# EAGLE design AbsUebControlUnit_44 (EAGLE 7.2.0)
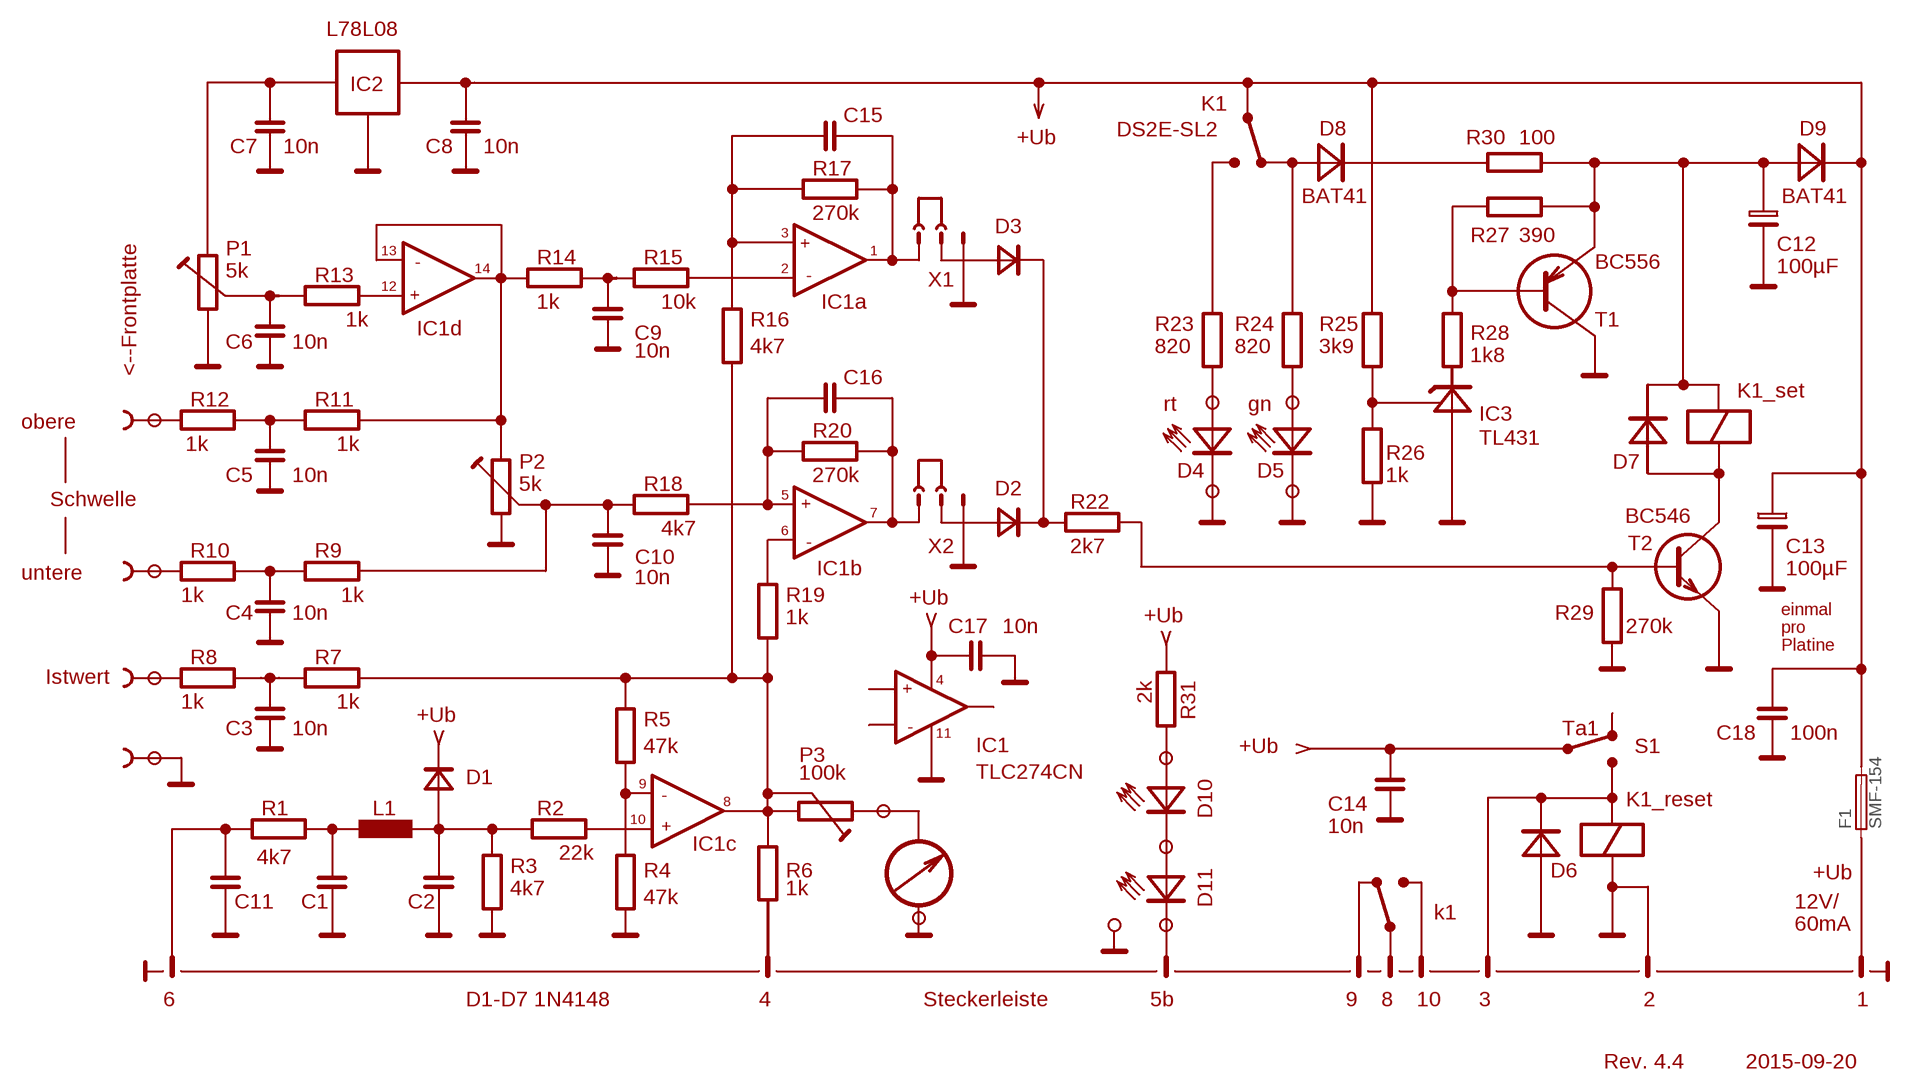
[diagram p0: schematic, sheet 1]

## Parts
F1  SMF-154  [SMF-154]
Unconnected: F1.1 F1.2

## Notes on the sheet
- L78L08
- IC2
- K1
- C15
- DS2E-SL2 | D8 | D9
- +Ub | R30 | 100
- C7 | 10n | C8 | 10n
- R17
- BAT41 | BAT41
- 270k
- D3
- 3 | +
- R27 | 390
- P1 | C12
- 13 | - | 1
- R14 | R15 | - | BC556
- 14 | 2 | 100µF
- 5k | R13
- X1
- 12
- +
- 1k | 10k | IC1a
- 1k | R16 | R23 | R24 | R25 | T1
- IC1d | C9 | R28
- C6 | 10n | 4k7 | 820 | 820 | 3k9
- 10n | 1k8
- <--Frontplatte
- C16
- K1_set
- R12 | R11 | rt | gn
- IC3
- obere
- R20
- TL431
- 1k | 1k
- R26
- P2 | D7
- C5 | 10n | 270k | D4 | D5 | 1k
- Schwelle | 5k | R18 | D2
- 5
- + | R22
- 7
- BC546
- 4k7 | 6 | - | T2
- C10 | X2 | 2k7 | C13
- R10 | R9
- untere | IC1b | 100µF
- 10n
- 1k | 1k | R19 | +Ub
- C4 | 10n | R29 | einmal
- 1k | +Ub
- C17 | 10n | 270k | pro
- Platine
- Istwert | R8 | R7
- 2k | R31
- 4
- +
- 1k | 1k
- +Ub | -
- R5
- C3 | 10n | 11 | Ta1 | C18 | 100n
- 47k | IC1 | +Ub | S1
- P3
- D1 | 100k | TLC274CN | D10
- 9 | -
- 8 | K1_reset
- R1 | L1 | R2 | C14
- +
- 10
- 10n
- IC1c
- 4k7 | 22k | +Ub
- R3 | D11
- R4 | R6 | D6
- 4k7 | 1k
- C11 | C1 | C2 | 47k | k1 | 12V/
- 60mA
- 6 | D1-D7 1N4148 | 4 | Steckerleiste | 5b | 9 | 8 | 10 | 3 | 2 | 1
- Rev. 4.4 | 2015-09-20

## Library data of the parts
F1 = AbsUebParts_11:SMF-154: Littelfuse Surface Mount Fuse; MF: Littelfuse; MPN: 154.250; OC_REICHELT: SMD-HASF 0,25A; OC_RS: 219-6068

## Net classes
0 default: clearance 0.205 mm

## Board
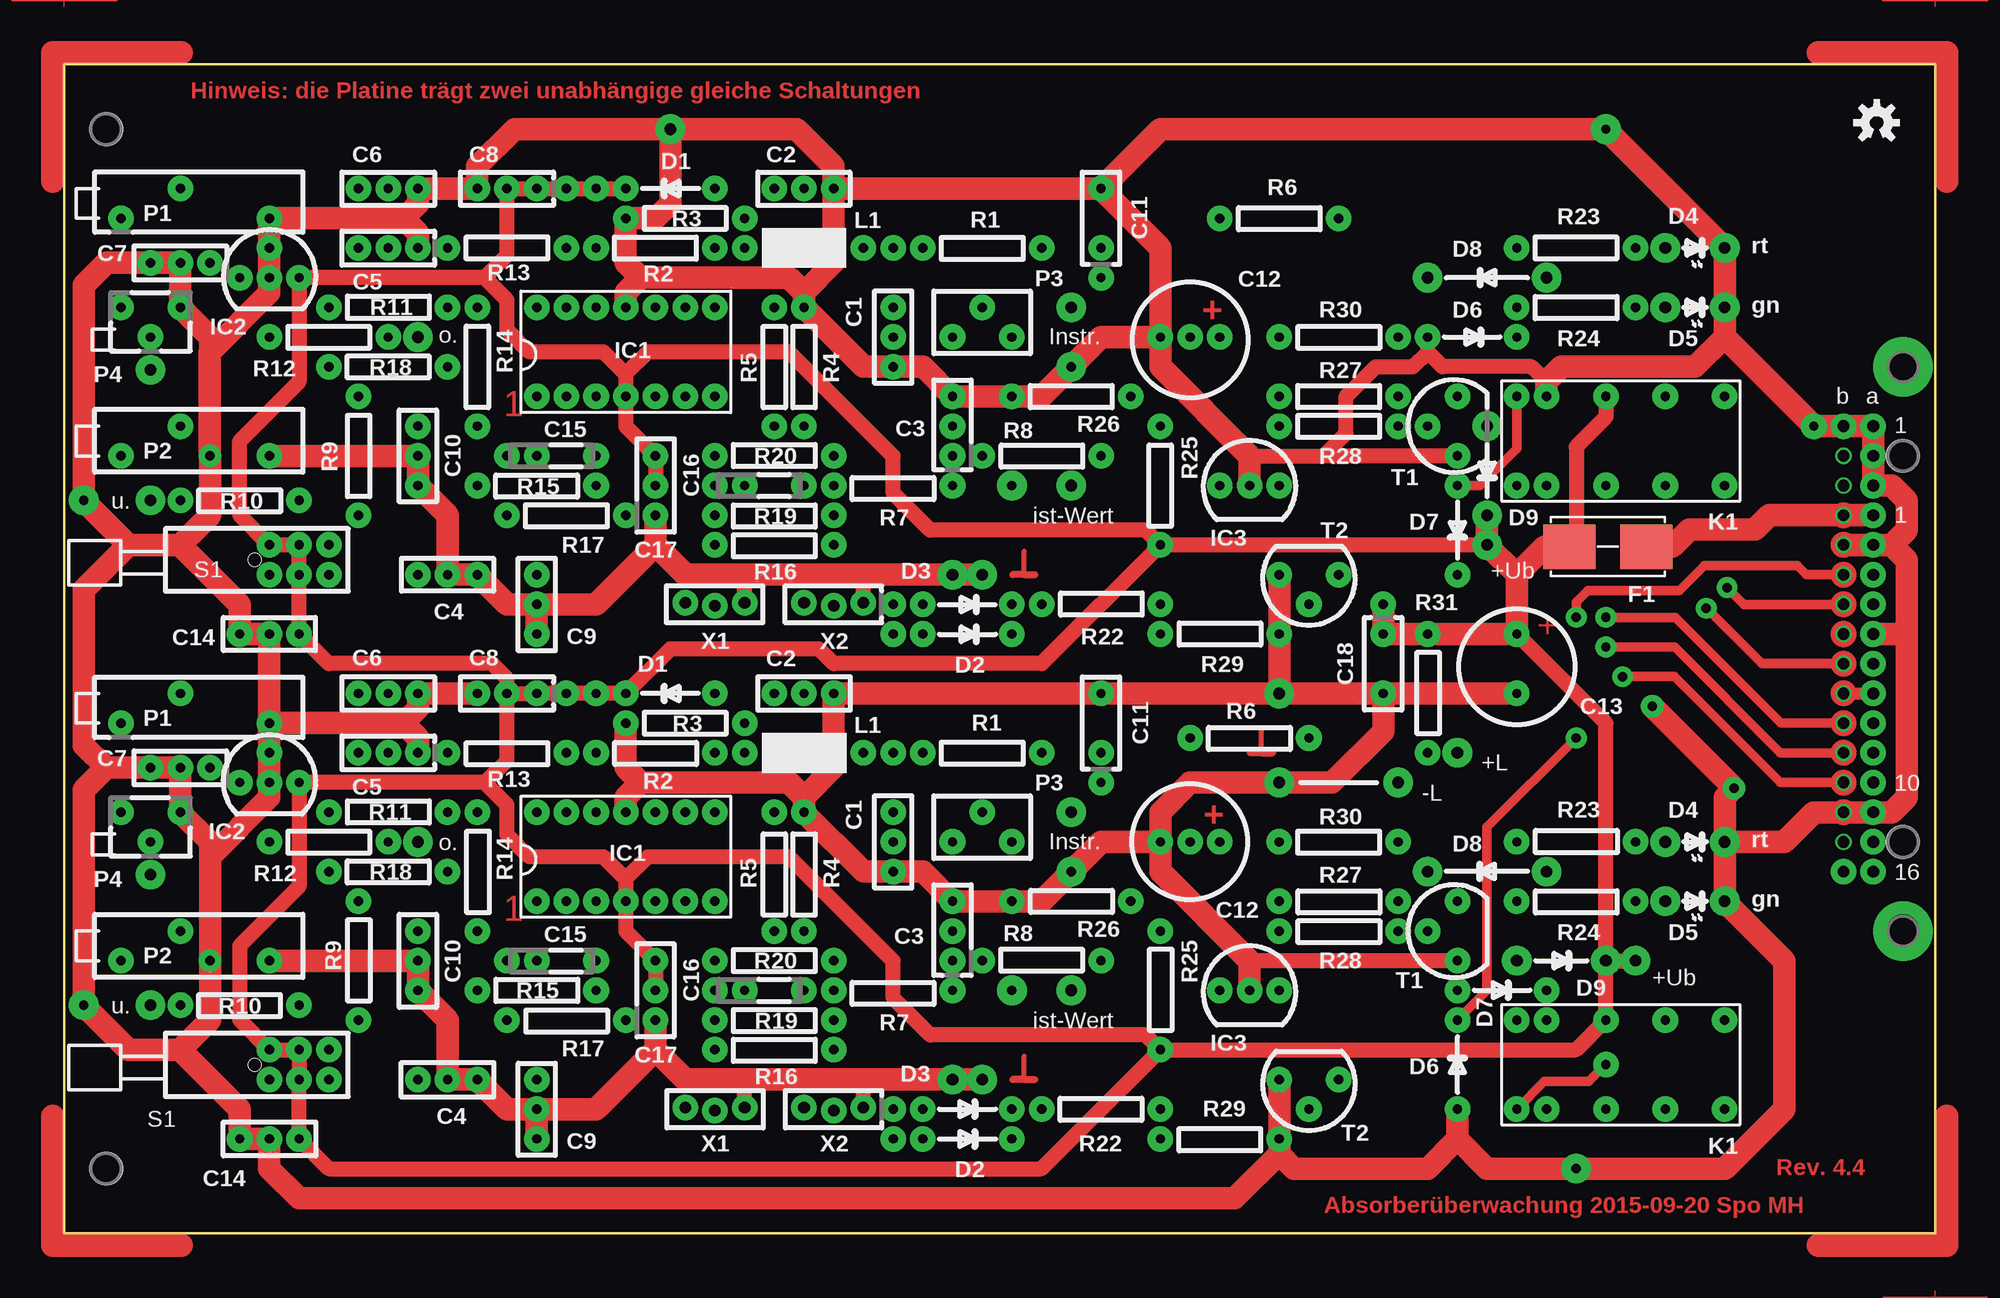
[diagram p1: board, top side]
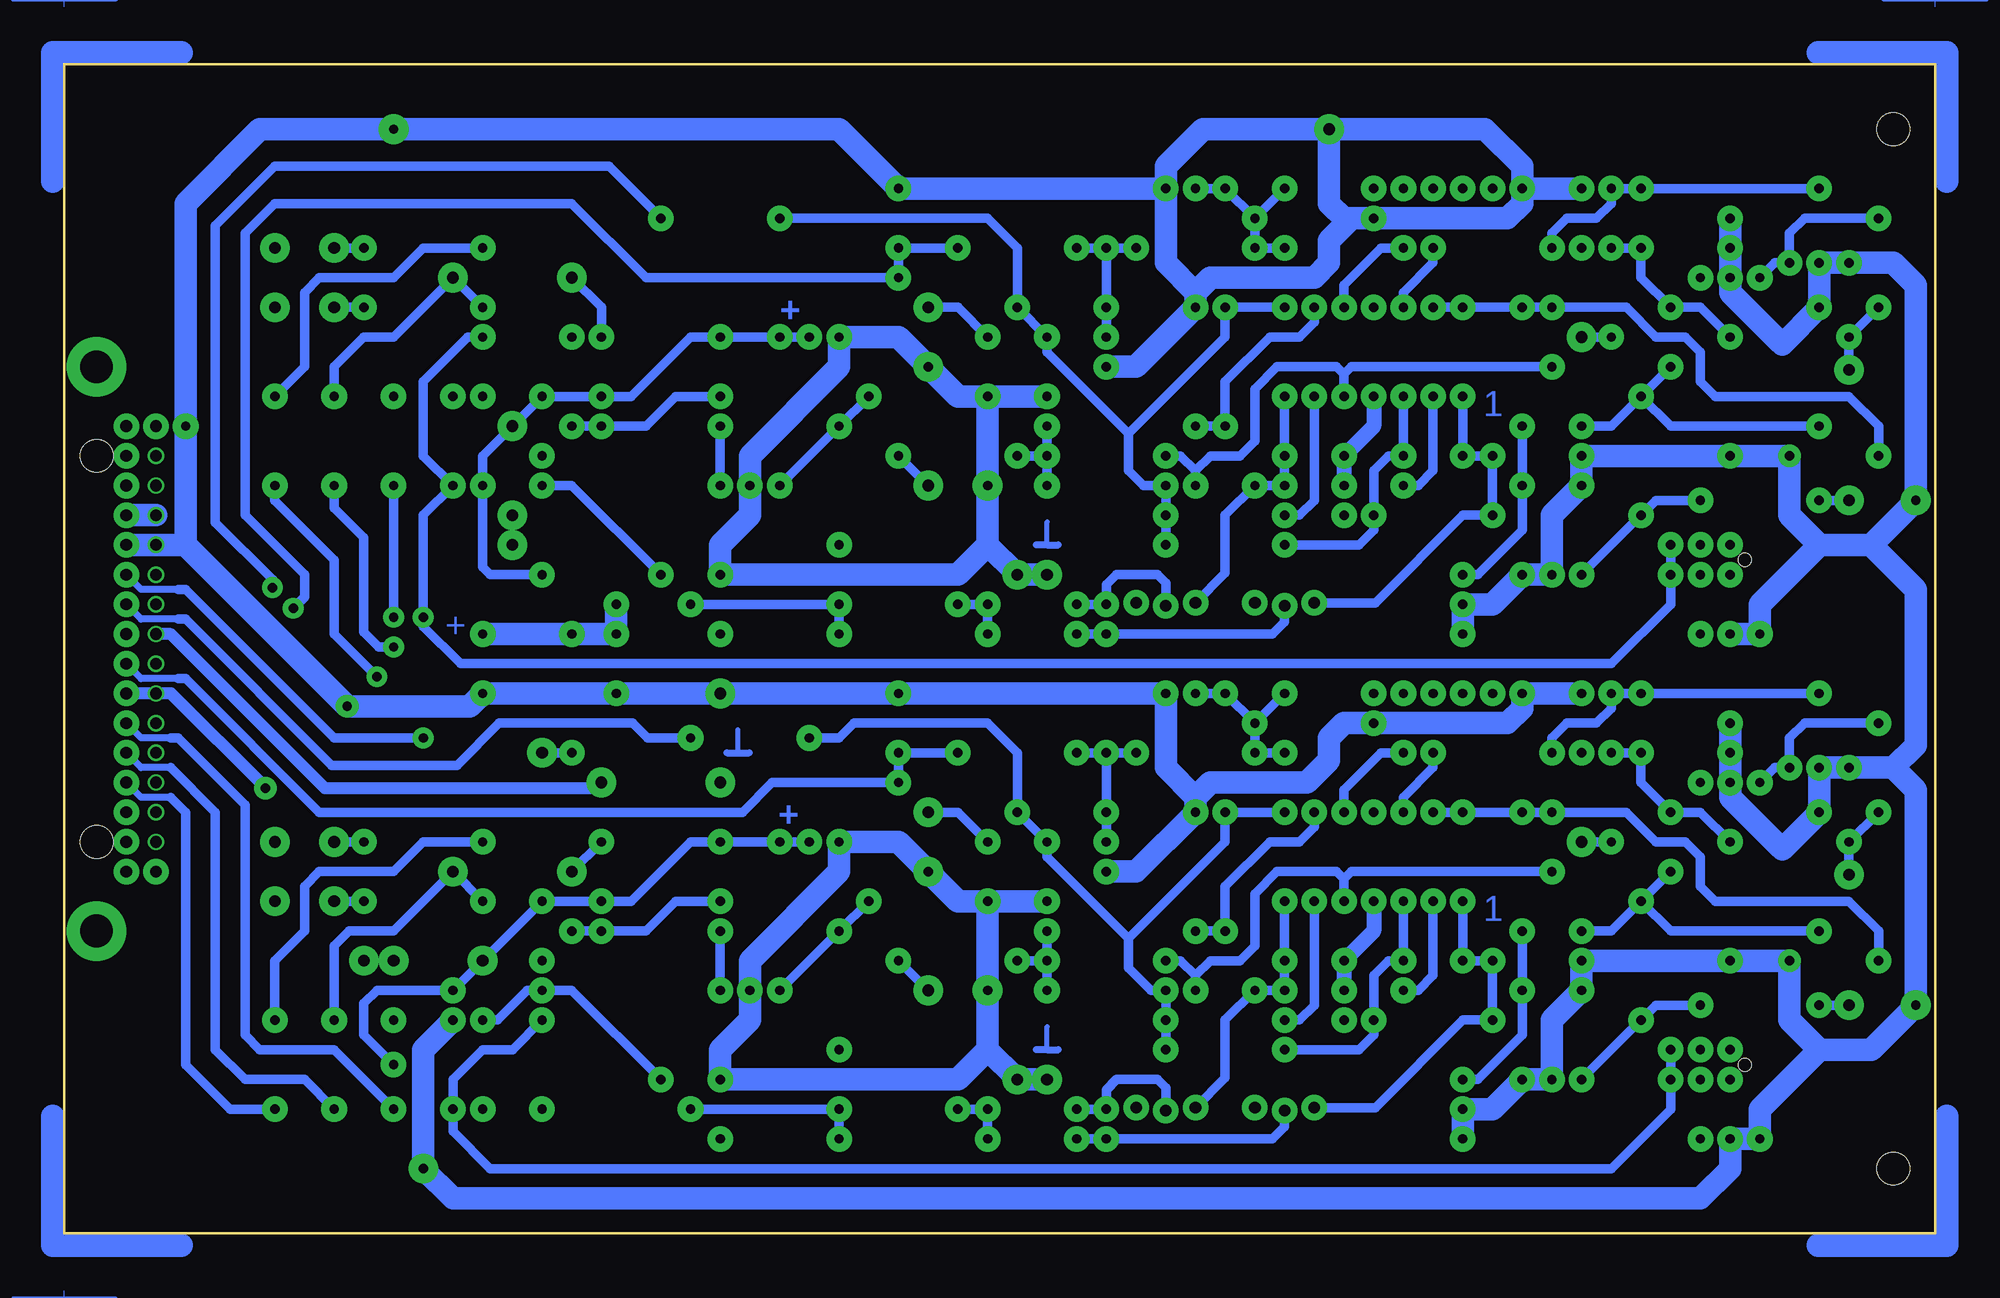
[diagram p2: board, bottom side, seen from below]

Size 160 x 100 mm. Coordinates in mm from the lower left corner, seen from the top.
Outline: 0,0 160,0 160,100 0,100 0,0
Copper layers (1*16): Top 0.035mm / dielectric 1.5mm / Bottom 0.035mm
Design rules "Aetzwerk-DRC 2 Lagen 35µm Cu": minimum track width 6mil, minimum drill 12mil, track to track 6mil, track to pad 6mil, pad to pad 6mil, via to via 6mil, smd to smd 6mil, copper to edge 20mil, drill to drill 8mil, minimum pad ring 8mil, minimum via ring 6mil, stop-mask expansion 3mil, vias tented up to drill 0mil, thermal gap 8mil
Holes 2.8 mm at 3.57,5.55 3.57,94.45 157.24,33.49 157.24,66.51
Holes 1.1 mm at 16.27,57.62 16.27,14.44
vRestrict: area 1.3,92.2 to 5.9,96.7; area 1.3,3.3 to 5.9,7.8; area 155,71.8 to 159.5,76.4; area 155,23.6 to 159.5,28.2

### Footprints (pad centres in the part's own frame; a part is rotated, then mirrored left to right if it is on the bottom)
SMF-154 = smd 4.445 x 3.81: 1 -3.289,0; 2 3.289,0

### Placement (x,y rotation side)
DRILEGEND  [DRILEGEND]  not placed on the board
F1  132,58.74 0 top
PM1  [PASSMARK]  not placed on the board
PM2  [PASSMARK]  not placed on the board
PM3  [PASSMARK]  not placed on the board

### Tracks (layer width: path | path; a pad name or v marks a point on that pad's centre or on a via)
+L  (via drill 0.8 pad 2.18, 1 pad 2.54)
  Bottom 0.813: v116.6,41.11 v119.14,41.11
+UB  (via drill 1 pad 1.4, 1 pad 2.18)
  Top 1.93: v154.7,61.43 v152.16,61.43 145.81,61.43 144.57,60.2 138.96,60.2 137.5,58.74 135.19,58.74
  Bottom 1.93: v152.16,61.43 v154.7,61.43
-L  (via drill 1 pad 1.4, 1 pad 2.54)
  Bottom 1.016: v152.16,51.27 150.89,51.27 137.72,38.1 114.53,38.1 v114.06,38.57
GND  (via drill 0.8 pad 1.93, 0.8 pad 2.18, 0.8 pad 2.54, 1 pad 1.4, 1 pad 2.18, 1 pad 2.54)
  Top 0.813: 58.18,13.17 58.42,13.17
  Top 1.016: v152.16,46.19 v154.7,46.19 | 157.56,51.27 157.56,50.8
  Top 1.27: 116.6,75.4 v116.6,76.67 | 116.6,75.4 117.87,74.13 125.49,74.13 126.76,72.86 | 116.6,75.4 115.33,74.13 112.16,74.13 109.61,71.59 109.61,68.42 107.71,66.51 | 101.36,66.51 107.71,66.51 | v119.14,66.51 107.71,66.51 | v119.14,23.33 101.36,23.33 | v58.18,10.76 58.18,13.17 | v68.34,10.76 68.34,13.17 68.58,13.17 | v58.18,53.94 58.18,56.35 58.42,56.35 | v68.34,53.94 68.34,56.35 67.94,56.35
  Top 1.93: 119.14,8.09 v119.14,10.63 | 119.14,8.09 121.68,5.55 v129.3,5.55 142,5.55 147.08,10.63 147.08,23.33 v142,28.41 v142,33.49 | 119.14,8.09 116.6,5.55 105.17,5.55 103.9,6.82 | v40.4,10.63 v40.4,8.09 | v126.76,71.59 126.76,72.86 128.03,74.13 139.46,74.13 142,76.67 | v101.36,20.79 101.36,23.33 93.74,30.95 v93.74,33.49 | 50.56,15.71 v50.56,18.25 | 50.56,15.71 53.1,13.17 58.42,13.17 68.58,13.17 v75.96,13.17 v78.5,13.17 | 103.9,6.82 v103.9,8.09 v103.9,13.17 | 156.29,58.89 157.56,60.16 157.56,62.7 156.29,63.97 v154.7,63.97 v154.7,66.51 v154.7,69.05 v152.16,69.05 v149.62,69.05 142,76.67 | 156.29,58.89 157.56,57.62 157.56,50.8 157.56,37.3 156.29,36.03 v154.7,36.03 v152.16,36.03 149.62,36.03 147.08,33.49 v142,33.49 | v142,33.49 142,37.3 v142.79,38.09 v135.81,45.08 | 156.29,58.89 v154.7,58.89 v152.16,58.89 | v93.74,33.49 93.74,36.03 96.28,38.57 v103.9,38.57 108.42,38.57 112.79,42.94 v112.79,46.19 | v93.74,33.49 88.66,33.49 v86.12,30.95 83.58,28.41 v81.04,28.41 v75.96,28.41 73.42,30.95 v70.88,30.95 68.34,30.95 v63.26,36.03 63.26,37.3 | 142,76.67 v142,79.21 v142,84.29 v131.84,94.45 93.74,94.45 v88.66,89.37 | v101.36,63.97 101.36,66.51 93.74,74.13 v93.74,76.67 | v93.74,76.67 88.66,76.67 v86.12,74.13 83.58,71.59 v81.04,71.59 v75.96,71.59 73.42,74.13 v70.88,74.13 68.34,74.13 v63.26,79.21 63.26,80.48 | v93.74,76.67 93.74,84.29 v88.66,89.37 | v112.79,46.19 v124.22,46.19 | 63.26,80.48 65.8,83.02 v65.8,89.37 | v103.9,56.35 v103.9,51.27 v103.9,46.19 | v48.02,79.21 48.02,80.48 49.29,81.75 | 63.26,80.48 61.99,81.75 49.29,81.75 | v65.8,89.37 v88.66,89.37 | v103.9,46.19 v112.79,46.19
  Top 1.93: v103.9,46.19 v88.66,46.19 v65.8,46.19 65.8,39.84 63.26,37.3 | v65.8,89.37 65.8,91.28 62.62,94.45 v51.83,94.45 | 49.29,81.75 48.02,83.02 v48.02,86.83 50.56,86.83 51.83,88.1 v51.83,94.45 | v78.5,56.35 v75.96,56.35 67.94,56.35 58.42,56.35 53.1,56.35 50.56,58.89 | v51.83,94.45 38.49,94.45 35.32,91.28 v35.32,89.37 v30.24,89.37 30.24,88.1 28.97,86.83 | v48.02,36.03 48.02,37.3 49.29,38.57 | 63.26,37.3 61.99,38.57 49.29,38.57 | 50.56,58.89 v50.56,61.43 | 50.56,58.89 45.48,53.81 v40.4,53.81 | 49.29,38.57 48.02,39.84 v48.02,43.65 | v40.4,53.81 v40.4,51.27 | v40.4,53.81 37.86,53.81 v35.32,56.35 v32.78,56.35 32.78,61.43 v30.24,63.97 v30.24,66.51 v17.54,66.51 | v30.24,84.29 30.24,85.56 28.97,86.83 | 28.97,86.83 v17.54,86.83 v17.54,84.29 17.54,80.48 12.46,75.4 12.46,76.67 9.92,79.21 9.92,83.02 v7.38,83.02 | v35.32,46.19 v30.24,46.19 30.24,44.92 28.97,43.65 | v30.24,41.11 30.24,42.38 28.97,43.65 | v17.54,43.65 28.97,43.65 | v12.46,66.51 12.46,61.43 9.92,58.89 | v17.54,43.65 v17.54,41.11 v17.54,38.57 17.54,37.3 12.46,32.22 | 5.47,58.89 9.92,58.89 | 5.47,58.89 v1.67,62.7 | 12.46,32.22 v12.46,23.33 12.46,18.25 9.92,15.71 | 5.47,58.89 1.67,55.08 1.67,41.74 3.57,39.84 | 3.57,39.84 v7.38,39.84 v9.92,39.84 v9.92,36.03 12.46,33.49 12.46,32.22 | 3.57,39.84 1.67,37.94 v1.67,19.52 5.47,15.71 9.92,15.71 | v40.4,10.63 37.86,10.63 v35.32,13.17 v32.78,13.17 32.78,18.25 v30.24,20.79 v30.24,23.33 v17.54,23.33 | v40.4,10.63 45.48,10.63 50.56,15.71 | 9.92,15.71 15,10.63 v15,8.09 v17.54,8.09 17.54,5.55 20.08,3.01 100.09,3.01 103.9,6.82 | v17.54,43.65 v17.54,51.27 v15,51.27 15,53.81 9.92,58.89 | v154.7,51.27 157.56,51.27
  Bottom 1.016: v154.7,46.19 v152.16,46.19 150.89,46.19 v142.79,38.09
  Bottom 1.93: v40.4,8.09 v40.4,10.63 37.86,10.63 v35.32,13.17 v32.78,13.17 32.78,18.25 v30.24,20.79 v30.24,23.33 v17.54,23.33 v12.46,23.33 12.46,18.25 9.92,15.71 | v75.96,13.17 v78.5,13.17 81.04,15.71 | v154.7,58.89 v152.16,58.89 149.62,58.89 | 149.62,58.89 v149.62,69.05 149.62,88.1 143.27,94.45 v131.84,94.45 93.74,94.45 v88.66,89.37 v65.8,89.37 | 81.04,15.71 83.58,13.17 v103.9,13.17 103.9,15.71 101.36,18.25 v101.36,20.79 101.36,23.33 93.74,30.95 v93.74,33.49 88.66,33.49 v86.12,30.95 83.58,28.41 v81.04,28.41 | 81.04,15.71 v81.04,20.79 v81.04,28.41 | 149.62,58.89 v135.81,45.08 125.33,45.08 v124.22,46.19 v112.79,46.19 v103.9,46.19 v88.66,46.19 v65.8,46.19 65.8,39.84 63.26,37.3 | v70.88,74.13 68.34,74.13 v63.26,79.21 63.26,80.48 | 63.26,80.48 61.99,81.75 53.1,81.75 51.83,83.02 51.83,84.92 49.92,86.83 | v81.04,28.41 v75.96,28.41 | 63.26,80.48 65.8,83.02 v65.8,89.37 | v81.04,71.59 83.58,71.59 v86.12,74.13 88.66,76.67 v93.74,76.67 93.74,74.13 101.36,66.51 v101.36,63.97 101.36,61.43 103.9,58.89 v103.9,56.35 83.58,56.35 81.04,58.89 | v81.04,71.59 v75.96,71.59 | v81.04,71.59 v81.04,63.97 81.04,58.89 | v65.8,89.37 65.8,91.28 62.62,94.45 v51.83,94.45 | 81.04,58.89 v78.5,56.35 v75.96,56.35 | 49.92,86.83 50.56,86.83 51.83,88.1 v51.83,94.45 | v70.88,30.95 68.34,30.95 v63.26,36.03 63.26,37.3 | 63.26,37.3 61.99,38.57 53.73,38.57 51.83,40.48 51.83,42.38 50.56,43.65 v48.02,43.65 36.59,43.65 35.32,44.92 v35.32,46.19 v30.24,46.19 | 49.92,86.83 v48.02,86.83 36.59,86.83 35.32,88.1 v35.32,89.37 | v51.83,94.45 38.49,94.45 35.32,91.28 v35.32,89.37 | v30.24,89.37 v35.32,89.37 | v40.4,51.27 v40.4,53.81 37.86,53.81 v35.32,56.35 v32.78,56.35 32.78,61.43 v30.24,63.97 v30.24,66.51 v17.54,66.51 v12.46,66.51 12.46,61.43 9.92,58.89
  Bottom 1.93: v17.54,86.83 v17.54,84.29 17.54,80.48 13.2,76.14 | v17.54,43.65 v17.54,41.11 v17.54,38.57 17.54,37.3 13.2,32.96 | 5.47,58.89 9.92,58.89 | 5.47,58.89 v1.67,62.7 | 5.47,58.89 1.67,55.08 1.67,41.74 3.57,39.84 | 3.57,39.84 v7.38,39.84 v9.92,39.84 v9.92,36.03 13.09,32.86 | 3.57,39.84 1.67,37.94 v1.67,19.52 5.47,15.71 9.92,15.71 | 9.92,15.71 15,10.63 v15,8.09 v17.54,8.09 17.54,5.55 20.08,3.01 126.76,3.01 v129.3,5.55 129.3,15.71 v126.76,18.25 | 9.92,58.89 15,53.81 v15,51.27 v17.54,51.27
N$1  (via drill 0.8 pad 1.78, 0.8 pad 2.18, 1 pad 1.4)
  Top 0.813: v152.16,56.35 148.99,56.35 148.19,57.15 140.25,57.15 138.11,55 130.3,55 129.3,54 v129.3,52.7
  Bottom 0.813: v124.22,76.67 125.49,76.67 129.3,72.86 129.3,66.51 v126.76,63.97 129.3,61.43 v129.3,52.7 129.3,51.91 126.12,48.73 27.7,48.73 22.62,53.81 v22.62,56.35 v22.62,58.89
N$2  (via drill 0.8 pad 2.18)
  Top 0.813: v124.22,71.59 124.22,67.14 121.05,63.97 v119.14,63.97
  Bottom 0.813: v108.98,56.35 116.6,63.97 v119.14,63.97
N$3  (via drill 2.8 pad 5.08)
  other vias: 157.24,74.13
N$4  (via drill 0.8 pad 1.78, 0.8 pad 2.18, 1 pad 2.18)
  Top 0.813: v129.3,42.38 121.68,34.76 121.68,20.79 v119.14,18.25
  Bottom 0.61: v154.7,56.35 153.43,55.08 150.25,55.08
  Bottom 0.813: v22.62,15.71 v22.62,13.17 22.62,10.63 27.7,5.55 123.58,5.55 126.76,8.72 v126.76,10.63 126.76,13.17 124.22,15.71 121.68,15.71 v119.14,18.25 | 150.25,55.08 149.62,55.08 136.92,42.38 v129.3,42.38
N$5  (via drill 0.8 pad 2.18)
  Bottom 0.813: v42.94,84.29 42.94,83.02 45.48,80.48 v45.48,79.21
N$6
  Top 1.93: 12.45,66.53 12.45,75.42
N$7  (via drill 0.8 pad 2.18, 1 pad 2.54)
  Bottom 0.813: v119.14,56.35 123.58,56.35 124.22,56.98 v124.22,63.97 124.22,66.51 v121.68,69.05 v119.14,71.59 v114.06,71.59 111.52,71.59 106.44,76.67 v103.9,76.67 v98.82,76.67 v96.28,76.67
N$8  (via drill 2.8 pad 5.08)
  other vias: 157.24,25.87
N$9  (via drill 0.8 pad 2.18, 1 pad 2.54)
  Top 0.813: v131.84,14.44 130.4,13 126.59,13 v124.22,10.63
  Bottom 0.813: v96.28,33.49 v98.82,33.49 v103.9,33.49 106.44,33.49 111.52,28.41 v114.06,28.41 v119.14,28.41 v124.22,23.33 v126.76,20.79 133.25,20.79 134.38,19.66 134.38,16.98 v131.84,14.44
N$10  (via drill 0.8 pad 2.18)
  Bottom 0.813: v108.98,13.17 116.6,20.79 v119.14,20.79 120.41,20.79 122.95,18.25 v124.22,18.25
N$11
  Bottom 1.93: 1.68,62.7 1.68,81.11 3.58,83.02 7.39,83.02
N$12
  Bottom 1.93: 6.92,83.02 9.92,83.02 9.92,79.21 13.09,76.04
N$13  (via drill 0.8 pad 2.18)
  other vias: 9.92,79.21
N$14  (via drill 0.8 pad 2.18, 1 pad 2.54)
  Bottom 0.813: v7.38,73.88 v7.38,76.67 v4.84,79.21
N$15
  Top 1.93: 7.39,83.02 3.58,83.02 1.68,81.11 1.68,62.7
N$16  (via drill 0.8 pad 2.18)
  other vias: 17.54,81.75
N$17  (via drill 0.8 pad 2.18)
  other vias: 9.92,83.02
N$18  (via drill 0.8 pad 2.18)
  Bottom 0.813: v15,81.75 13.73,83.02 v12.46,83.02
N$19  (via drill 0.8 pad 2.18)
  other vias: 42.94,41.11
N$20  (via drill 0.8 pad 2.18)
  Bottom 0.813: v15,38.57 13.73,39.84 v12.46,39.84 12.46,42.36 11.17,43.65 v4.84,43.65
N$21  (via drill 0.8 pad 2.18, 1 pad 2.54)
  Bottom 0.813: v7.38,33.49 v7.38,30.7
N$22  (via drill 0.8 pad 2.18)
  Bottom 0.813: v4.84,36.03 7.38,33.49
N$23  (via drill 0.8 pad 2.18)
  other vias: 4.84,86.83
N$24
  Bottom 0.813: 42.94,41.11 42.94,39.84 45.48,37.3 45.48,36.03
N$25
  Top 2: 10,101 -1,101 -1,90
N$26
  Bottom 2: 10,101 -1,101 -1,90
N$27
  Top 2: 10,-1 -1,-1 -1,10
N$28
  Bottom 2: 10,-1 -1,-1 -1,10
N$29
  Top 2: 150,-1 161,-1 161,10
N$30
  Bottom 2: 150,-1 161,-1 161,10
N$31
  Top 2: 161,90 161,101 150,101
N$32
  Bottom 2: 161,90 161,101 150,101
N$33  (via drill 1 pad 2.18)
  other vias: 152.16,30.95
N$34
  Bottom 0.813: 4.84,86.83 11.17,86.83 12.46,85.54 12.46,83.02
N$35  (via drill 0.8 pad 2.18, 1 pad 2.18)
  Bottom 0.813: v73.42,8.09 v70.88,8.09 56.68,8.09 55.64,9.13 v55.64,10.5
N$36  (via drill 0.8 pad 2.18, 1 pad 2.18)
  Bottom 0.813: v73.42,10.63 v70.88,10.63 70.88,12.3 70.02,13.17 66.51,13.17 65.8,12.46 v65.8,10.5
N$38  (via drill 0.8 pad 2.18, 1 pad 2.18)
  Bottom 0.813: v73.42,53.81 v70.88,53.81 70.88,55.48 70.02,56.35 66.51,56.35 65.8,55.64 v65.8,53.68
N$39  (via drill 0.8 pad 2.18, 1 pad 2.18)
  Bottom 0.813: v73.42,51.27 v70.88,51.27 56.68,51.27 55.64,52.31 v55.64,53.68
S$1  (via drill 1 pad 1.4)
  other vias: 152.16,63.97
S$2  (via drill 0.8 pad 2.18, 1 pad 2.54)
  Bottom 0.813: v30.24,76.67 v27.7,76.67
S$3  (via drill 0.8 pad 2.18)
  Bottom 0.813: v63.26,25.87 v60.72,25.87 60.72,29.68 56.91,33.49 54.37,33.49 53.1,34.76 v53.1,36.03
S$4  (via drill 0.8 pad 2.18, 1 pad 2.54)
  Bottom 0.813: v81.04,33.49 83.58,36.03 v86.12,36.03
S$5  (via drill 0.8 pad 2.18)
  Bottom 0.813: v22.62,79.21 20.08,79.21 v17.54,76.67
S$6
  Bottom 0.813: 12.46,83.02 13.73,83.02
S$7  (via drill 0.8 pad 2.18)
  other vias: 17.54,13.17
S$8  (via drill 0.8 pad 2.18)
  Bottom 0.813: v45.48,63.97 44.21,63.97 42.94,65.24 v42.94,71.59
S$9  (via drill 1 pad 1.4)
  other vias: 152.16,66.51
S$10  (via drill 0.8 pad 2.18, 1 pad 2.18)
  Bottom 0.61: v154.7,38.57 153.43,37.3 150.89,37.3
  Bottom 0.813: v142,10.63 145.81,10.63 149.62,14.44 149.62,36.03 150.89,37.3
S$11  (via drill 0.8 pad 2.18)
  Bottom 0.813: v70.88,41.11 v68.34,41.11 | v70.88,41.11 v73.42,41.11 | v70.88,33.49 v70.88,36.03 v70.88,41.11
S$12
  Bottom 0.406: 75.96,58.9 75.96,60.88
  Bottom 0.61: 74.99,58.9 75.96,58.9 76.89,58.9
S$18  (via drill 0.8 pad 2.18, 1 pad 2.18)
  Bottom 0.61: v154.7,43.65 153.43,42.38 150.89,42.38
  Bottom 0.813: v131.84,10.63 136.92,15.71 143.27,15.71 144.54,16.98 144.54,36.66 150.25,42.38 150.89,42.38
S$19  (via drill 0.8 pad 2.18, 1 pad 2.18)
  Bottom 0.61: v154.7,41.11 153.43,39.84 150.89,39.84
  Bottom 0.813: v136.92,10.63 139.46,13.17 144.54,13.17 147.08,15.71 147.08,36.03 150.89,39.84
S$20  (via drill 0.8 pad 2.18)
  Bottom 0.813: v20.08,19.52 23.89,19.52 v25.16,18.25 v30.24,13.17
S$21  (via drill 0.8 pad 2.18)
  Bottom 0.813: 50.56,30.32 v50.56,28.41 | 50.56,30.32 51.2,30.95 56.27,30.95 58.18,29.05 58.18,24.6 59.45,23.33 61.99,23.33 63.26,22.06 | 50.56,30.32 49.92,30.95 v32.78,30.95 | v65.8,23.33 64.53,23.33 63.26,22.06 | 63.26,22.06 v63.26,20.79
S$22  (via drill 0.8 pad 2.18, 1 pad 2.18)
  Bottom 0.813: v55.64,71.59 v55.64,66.51 v55.64,63.97 v58.18,63.97 60.72,61.43 60.72,56.48 v63.26,53.94
S$23  (via drill 0.8 pad 2.18)
  Bottom 0.813: v45.48,71.59 v45.48,66.51 46.75,66.51 48.02,65.24 v48.02,61.43 48.02,60.16 49.29,58.89 v55.64,58.89
S$24  (via drill 0.8 pad 2.18, 1 pad 2.18)
  Bottom 0.813: v40.4,71.59 v40.4,66.51 v37.86,66.51 v37.86,61.43 40.4,61.43 47.89,53.94 v53.1,53.94
S$25  (via drill 0.8 pad 2.18, 1 pad 2.18)
  Bottom 0.813: v55.64,28.41 v55.64,23.33 v55.64,20.79 v58.18,20.79 60.72,18.25 60.72,13.3 v63.26,10.76
S$26  (via drill 1 pad 2.18)
  other vias: 154.7,33.49
S$28  (via drill 0.8 pad 2.18)
  Bottom 0.813: v42.94,79.21 v40.4,79.21 v35.32,79.21 v32.78,79.21 26.43,79.21 23.89,76.67 21.35,76.67 20.08,75.4 20.08,72.86 18.81,71.59 7.38,71.59 4.84,69.05 v4.84,66.51
S$29  (via drill 1 pad 2.18)
  other vias: 154.7,30.95
S$30  (via drill 0.8 pad 2.18)
  Bottom 0.813: v55.64,61.43 54.37,61.43 53.1,62.7 v53.1,71.59
S$32  (via drill 0.8 pad 2.18)
  Bottom 0.813: v35.32,69.05 v35.32,63.97 35.32,60.16 39.13,56.35 v40.4,56.35
S$34  (via drill 0.8 pad 2.18, 1 pad 2.18)
  Bottom 0.813: v40.4,28.41 v40.4,23.33 v37.86,23.33 v37.86,18.25 40.4,18.25 47.89,10.76 v53.1,10.76
S$35  (via drill 0.8 pad 2.18)
  Bottom 0.813: v83.58,53.81 v81.04,53.81 v81.04,51.27
S$38  (via drill 1 pad 1.4)
  other vias: 152.16,33.49
S$39
  Top 0.406: 102.4,41.12 102.4,43.1
  Top 0.61: 101.43,41.12 102.4,41.12 103.33,41.12
S$41
  Top 0.406: 82.08,13.18 82.08,15.16
  Top 0.61: 81.11,13.18 82.08,13.18 83.01,13.18
S$42
  Top 0.406: 82.08,56.35 82.08,58.34
  Top 0.61: 81.11,56.35 82.08,56.35 83.01,56.35
S$43  (via drill 0.8 pad 2.18)
  Bottom 0.813: v142,18.25 142,23.33 139.46,25.87 139.46,29.68 138.19,30.95 131.84,30.95 129.3,33.49 v124.22,33.49
S$44  (via drill 0.8 pad 2.18)
  Bottom 0.813: v106.44,10.63 v93.74,10.63 v93.74,8.09
S$45  (via drill 0.8 pad 2.18, 1 pad 2.54)
  Bottom 0.813: v134.38,33.49 v136.92,33.49
S$46  (via drill 0.8 pad 2.18)
  Bottom 0.813: v45.48,28.41 v45.48,23.33 46.75,23.33 48.02,22.06 v48.02,18.25 48.02,16.98 49.29,15.71 v55.64,15.71
S$48  (via drill 0.8 pad 2.18)
  Bottom 0.813: v45.48,20.79 44.21,20.79 42.94,22.06 v42.94,28.41
S$51
  Bottom 0.406: 75.96,15.71 75.96,17.7
  Bottom 0.61: 74.99,15.71 75.96,15.71 76.89,15.71
S$54  (via drill 0.8 pad 2.18)
  Bottom 0.813: v45.48,41.11 47.38,41.11 50.56,37.94 v50.56,36.03
S$56  (via drill 0.8 pad 2.18)
  Bottom 0.813: v55.64,18.25 54.37,18.25 53.1,19.52 v53.1,28.41
S$57  (via drill 0.8 pad 2.18, 1 pad 2.54)
  Bottom 0.813: v114.06,33.49 v116.6,30.95
S$60
  Bottom 0.406: 102.4,41.2 102.4,43.1
S$62
  Bottom 0.61: 103.33,41.12 101.43,41.12
S$66  (via drill 0.8 pad 2.18)
  other vias: 17.54,56.35
S$67  (via drill 0.8 pad 2.18)
  other vias: 45.48,36.03
S$68  (via drill 0.8 pad 2.18)
  Bottom 0.813: v42.94,36.03 v40.4,36.03 v35.32,36.03 v32.78,36.03 26.43,36.03 23.89,33.49 21.35,33.49 20.08,32.22 20.08,29.68 18.81,28.41 7.38,28.41 4.84,25.87 v4.84,23.33
S$69  (via drill 0.8 pad 2.18, 1 pad 2.54)
  Bottom 0.813: v7.38,62.7 v9.92,62.7
S$71  (via drill 0.8 pad 2.18)
  Bottom 0.813: v9.92,46.19 v25.16,46.19 v27.7,46.19 27.7,44.92 28.97,43.65 31.51,43.65 32.78,42.38 v32.78,41.11
S$73  (via drill 0.8 pad 2.18)
  Bottom 0.813: v35.32,25.87 v35.32,20.79 35.32,16.98 39.13,13.17 v40.4,13.17
S$76  (via drill 0.8 pad 2.18)
  Bottom 0.813: v83.58,10.63 v81.04,10.63 v81.04,8.09
S$79  (via drill 0.8 pad 2.18)
  Bottom 0.813: v50.56,79.21 50.56,81.11 47.38,84.29 v45.48,84.29
S$85  (via drill 0.8 pad 2.18, 1 pad 2.54)
  Bottom 0.813: v7.38,19.52 v9.92,19.52
S$86  (via drill 0.8 pad 2.18, 1 pad 2.54)
  Bottom 0.813: v88.66,66.51 v86.12,63.97
S$100  (via drill 0.8 pad 2.18)
  Bottom 0.813: v17.54,33.49 20.08,36.03 v22.62,36.03 25.16,38.57 v25.16,41.11 v27.7,41.11
S$101  (via drill 0.8 pad 2.18, 1 pad 2.54)
  Bottom 0.813: v30.24,33.49 v27.7,33.49
S$102  (via drill 0.8 pad 2.18)
  Bottom 0.813: 50.56,73.5 v50.56,71.59 | 50.56,73.5 51.2,74.13 56.27,74.13 58.18,72.22 58.18,67.78 59.45,66.51 61.99,66.51 63.26,65.24 | 50.56,73.5 49.92,74.13 v32.78,74.13 | v65.8,66.51 64.53,66.51 63.26,65.24 | 63.26,65.24 v63.26,63.97
S$105  (via drill 0.8 pad 1.78, 0.8 pad 2.18, 1 pad 1.4)
  Top 0.813: v152.16,48.73 145.17,48.73 v140.42,53.48
  Bottom 0.813: v83.58,84.29 v88.66,84.29 v88.66,81.75 110.25,81.75 116.6,88.1 142,88.1 144.54,85.56 144.54,61.43 139.46,56.35 139.46,54.44 v140.42,53.48
S$106  (via drill 0.8 pad 2.18)
  Bottom 0.813: v63.26,46.19 v60.72,46.19 v58.18,43.65 | v58.18,43.65 v55.64,46.19 | v55.64,41.11 v58.18,41.11 v58.18,43.65
S$108  (via drill 0.8 pad 2.18, 1 pad 2.18)
  Bottom 0.61: v154.7,53.81 153.43,52.54 150.25,52.54
  Bottom 0.813: 150.25,52.54 149.62,52.54 137.12,40.04 126.42,40.04 122.81,43.65 111.38,43.65 110.11,42.38 v106.44,42.38
S$110  (via drill 0.8 pad 2.18)
  Bottom 0.813: v75.96,23.33 v75.96,25.87 | v75.96,20.79 v75.96,23.33 | v75.96,23.33 v78.5,23.33
S$113  (via drill 0.8 pad 2.18)
  Bottom 0.813: v98.82,20.79 v93.74,25.87 v91.2,28.41
S$115  (via drill 0.8 pad 2.18, 1 pad 2.54)
  Bottom 0.813: v86.12,20.79 v88.66,23.33
S$116  (via drill 0.8 pad 2.18)
  Bottom 0.813: v55.64,36.03 v60.72,36.03 60.72,33.49 68.97,25.23 | 68.97,25.23 68.97,22.7 67.07,20.79 v65.8,20.79 v65.8,18.25 v65.8,15.71 | v96.28,42.38 93.74,42.38 92.47,43.65 81.04,43.65 78.5,41.11 v78.5,36.03 v75.96,33.49 75.96,32.22 68.97,25.23
S$119  (via drill 0.8 pad 2.18)
  Bottom 0.813: 22.62,79.21 25.16,81.75 v25.16,84.29 v27.7,84.29
S$121  (via drill 0.8 pad 2.18, 1 pad 2.18)
  Bottom 0.61: v154.7,48.73 153.43,47.46 150.25,47.46
  Bottom 0.813: 150.25,47.46 149.62,47.46 138.19,36.03 102,36.03 99.45,38.57 v88.66,38.57 v88.66,41.11 v83.58,41.11
S$122  (via drill 0.8 pad 2.18)
  Bottom 0.813: v30.24,25.87 27.7,25.87 v25.16,28.41 | v25.16,28.41 v22.62,30.95 | v25.16,28.41 22.62,25.87 v9.92,25.87
S$124  (via drill 0.8 pad 1.78, 0.8 pad 2.18, 1 pad 1.4)
  Top 0.813: v142.2,55.24 143.63,53.81 v152.16,53.81
  Bottom 0.813: v108.98,86.83 113.42,91.28 142,91.28 147.08,86.19 147.08,60.8 142.2,55.91 v142.2,55.24
S$132  (via drill 0.8 pad 2.18)
  Bottom 0.813: v103.9,63.97 v103.9,69.05
S$136  (via drill 0.8 pad 2.18)
  Bottom 0.813: v75.96,63.97 v75.96,66.51 | v75.96,66.51 v75.96,69.05 | v75.96,66.51 v78.5,66.51
S$137  (via drill 0.8 pad 2.18)
  Bottom 0.813: v63.26,69.05 v60.72,69.05 60.72,72.86 56.91,76.67 54.37,76.67 53.1,77.94 v53.1,79.21
S$142  (via drill 0.8 pad 2.18)
  Bottom 0.813: v70.88,84.29 v73.42,84.29 | v70.88,84.29 v68.34,84.29 | v70.88,76.67 v70.88,79.21 v70.88,84.29
S$143  (via drill 0.8 pad 2.18)
  Bottom 0.813: v103.9,71.59 107.71,71.59 110.25,69.05 v114.06,69.05 v116.6,69.05
S$144  (via drill 0.8 pad 2.18, 1 pad 2.54)
  Bottom 0.813: v114.06,76.67 114.06,79.21 v116.6,81.75
S$145  (via drill 0.8 pad 2.18)
  Bottom 0.813: v103.9,28.41 107.71,28.41 110.25,25.87 v114.06,25.87 v116.6,25.87
S$147  (via drill 0.8 pad 2.18, 1 pad 2.54)
  Bottom 0.813: v136.92,18.25 136.92,24.6 135.65,25.87 131.84,25.87 v126.76,30.95 v124.22,28.41
S$148  (via drill 0.8 pad 2.18)
  Bottom 0.813: v103.9,20.79 v103.9,25.87
S$149  (via drill 0.8 pad 2.18, 1 pad 2.54)
  Bottom 0.813: v134.38,28.41 v136.92,28.41
S$151  (via drill 0.8 pad 2.18)
  Bottom 0.813: v55.64,79.21 v60.72,79.21 60.72,76.67 68.97,68.42 | 68.97,68.42 68.97,65.24 67.7,63.97 v65.8,63.97 v65.8,61.43 v65.8,58.89 | v98.82,86.83 81.04,86.83 78.5,84.29 v78.5,79.21 v75.96,76.67 75.96,75.4 68.97,68.42
S$152  (via drill 0.8 pad 2.18)
  Bottom 0.813: v63.26,89.37 v60.72,89.37 v58.18,86.83 | v55.64,84.29 v58.18,84.29 v58.18,86.83 | v58.18,86.83 v55.64,89.37
S$155  (via drill 0.8 pad 2.18, 1 pad 2.54)
  Bottom 0.813: v81.04,76.67 83.58,79.21 v86.12,79.21
S$157  (via drill 0.8 pad 2.18)
  Bottom 0.813: v91.2,71.59 v93.74,69.05 v98.82,63.97
S$158  (via drill 0.8 pad 2.18)
  Bottom 0.813: v9.92,89.37 v25.16,89.37 v27.7,89.37 27.7,88.1 28.97,86.83 31.51,86.83 32.78,85.56 v32.78,84.29
S$159  (via drill 0.8 pad 2.18)
  Bottom 0.813: v106.44,53.81 v93.74,53.81 v93.74,51.27
S$160  (via drill 0.8 pad 2.18)
  Bottom 0.813: v20.08,62.7 23.89,62.7 v25.16,61.43 v30.24,56.35
S$161  (via drill 0.8 pad 2.18)
  Bottom 0.813: v30.24,69.05 27.7,69.05 v25.16,71.59 | v25.16,71.59 v22.62,74.13 | v25.16,71.59 22.62,69.05 v9.92,69.05
S$169  (via drill 0.8 pad 1.78, 0.8 pad 2.18, 1 pad 1.4)
  Top 0.813: v152.16,41.11 146.78,41.11 137.72,50.16 v131.84,50.16
  Bottom 0.813: v136.92,63.97 136.92,62.06 134.38,59.52 134.38,51.43 133.11,50.16 v131.84,50.16
S$170  (via drill 0.8 pad 1.78, 0.8 pad 2.18, 1 pad 1.4)
  Top 0.813: v152.16,43.65 146.81,43.65 137.76,52.7 v131.84,52.7
  Bottom 0.813: v131.84,52.7 v131.84,63.97
S$171  (via drill 0.8 pad 1.78, 0.8 pad 2.18, 1 pad 1.4)
  Top 0.813: v152.16,38.57 146.74,38.57 137.69,47.62 v133.27,47.62
  Bottom 0.813: v142,63.97 142,62.7 136.92,57.62 136.92,51.27 v133.27,47.62
S$172  (via drill 0.8 pad 2.18)
  Bottom 0.813: v142,71.59 139.46,74.13 139.46,80.48 138.19,81.75 131.84,81.75 129.3,84.29 v124.22,84.29
S$173  (via drill 0.8 pad 2.18, 1 pad 2.54)
  Bottom 0.813: v134.38,79.21 v136.92,79.21
S$177  (via drill 0.8 pad 2.18, 1 pad 2.54)
  Bottom 0.813: v134.38,84.29 v136.92,84.29
S$178  (via drill 0.8 pad 2.18, 1 pad 2.54)
  Bottom 0.813: v124.22,79.21 v126.76,81.75 131.84,76.67 134.38,76.67 136.92,74.13 v136.92,71.59
V+  (via drill 0.8 pad 2.18, 1 pad 2.54)
  Top 1.27: v48.02,89.37 v45.48,89.37 v42.94,89.37 v40.4,89.37 v37.86,89.37 37.86,83.66 35.95,81.75 | 35.95,81.75 v20.08,81.75 20.08,72.86 15,67.78 15,61.43 v17.54,58.89 v20.08,58.89 v20.08,56.35 v20.08,51.27 22.62,48.73 36.59,48.73 37.86,47.46 v37.86,46.19 | 35.95,81.75 37.86,79.84 37.86,77.31 39.77,75.4 46.12,75.4 48.02,73.5 | v50.56,63.97 v50.56,66.51 48.02,69.05 v48.02,71.59 48.02,73.5 | 48.02,73.5 49.92,75.4 61.99,75.4 70.88,66.51 70.88,63.34 74.06,60.16 92.47,60.16 v93.74,58.89 | v37.86,46.19 v40.4,46.19 v42.94,46.19 v45.48,46.19 v48.02,46.19 51.83,50 64.53,50 65.8,48.73 83.58,48.73 v93.74,58.89 | v37.86,46.19 37.86,40.48 35.95,38.57 | 35.95,38.57 v20.08,38.57 20.08,29.68 15,24.6 15,18.25 v17.54,15.71 v20.08,15.71 v20.08,13.17 v20.08,8.09 22.62,5.55 83.58,5.55 v93.74,15.71 | 35.95,38.57 37.86,36.66 37.86,34.12 39.77,32.22 46.12,32.22 48.02,30.32 | v50.56,20.79 v50.56,23.33 48.02,25.87 v48.02,28.41 48.02,30.32 | v121.68,58.89 v93.74,58.89 | 48.02,30.32 49.92,32.22 61.99,32.22 70.88,23.33 70.88,20.16 74.06,16.98 92.47,16.98 v93.74,15.71 | v124.22,51.27 131.84,43.65 v131.84,23.33 | v131.84,23.33 v131.84,18.25 129.3,15.71 v93.74,15.71 | v131.84,23.33 v134.38,23.33 | v131.84,71.59 131.84,69.84 129.3,67.3 129.3,58.74 128.81,58.74
  Top 1.93: 124.22,56.35 v121.68,58.89 v121.68,61.43 | 124.22,56.35 v124.22,51.27 v116.6,51.27 v112.79,51.27 v112.79,53.81 | 124.22,56.35 126.61,58.74 128.81,58.74
  Bottom 1.27: v50.56,63.97 v50.56,66.51 48.02,69.05 v48.02,71.59 | v50.56,20.79 v50.56,23.33 48.02,25.87 v48.02,28.41
  Bottom 1.93: v112.79,53.81 v112.79,51.27 v116.6,51.27 v124.22,51.27
(copper drawn outside any net)
  shapes: Top circle x11

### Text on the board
Top: Hinweis: die Platine trägt zwei unabhängige gleiche Schaltungen | + | 1 | + | + | 1 | Rev. 4.4 | Absorberüberwachung 2015-09-20 Spo MH
Bottom: + | 1 | + | + | 1
tPlace: P4 | P4
tNames: C6 | C8 | C2 | D1 | R6 | P1 | R3 | L1 | R1 | R23 | D4 | C11 | D8 | rt | C7 | R13 | C5 | R2 | P3 | C12 | R11 | gn | C1 | R30 | D6 | IC2 | o. | Instr. | R24 | D5 | IC1 | R5 | R4 | R14 | R12 | R18 | R27 | b | a | R26 | C15 | C3 | R8 | R25 | 1 | P2 | R20 | R28 | R9 | C10 | T1 | R15 | C16 | u. | R10 | R19 | R7 | ist-Wert | D9 | 1 | D7 | K1 | IC3 | T2 | R17 | C17 | S1 | R16 | D3 | +Ub | R31 | C4 | C14 | C9 | X1 | X2 | R22 | C6 | C8 | D1 | C2 | D2 | R29 | C18 | R6 | C13 | P1 | R3 | L1 | R1 | C11 | C7 | +L | C5 | R13 | R2 | P3 | 10 | -L | R23 | D4 | R11 | R30 | IC2 | C1 | o. | Instr. | D8 | rt | IC1 | R5 | R4 | R12 | R18 | R14 | R27 | 16 | gn | C12 | C15 | C3 | R8 | R26 | R25 | R24 | D5 | P2 | R20 | R28 | R9 | C10 | T1 | +Ub | R15 | C16 | D9 | u. | R10 | ist-Wert | D7 | R19 | R7 | IC3 | R17 | C17 | D6 | R16 | D3 | R29 | S1 | C4 | T2 | C9 | X1 | X2 | R22 | K1 | D2 | C14
DrillLegend: LAYER-STACK
DrillLegend_01-16: 01-16
DrillLegend_01-20: 01-20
